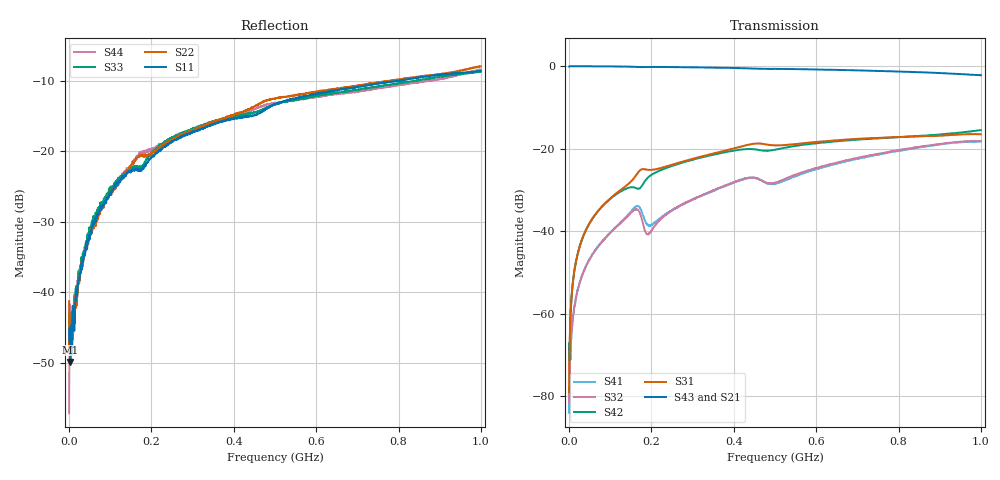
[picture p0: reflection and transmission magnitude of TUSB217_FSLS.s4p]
!Agilent Technologies,N5230A,US43500443,A.07.50.67
!Agilent N5230A: A.07.50.67
!Date: Wednesday, December 05, 2018 10:57:58
!Correction: S11(Full 4 Port(1,2,3,4))
!S12(Full 4 Port(1,2,3,4))
!S13(Full 4 Port(1,2,3,4))
!S14(Full 4 Port(1,2,3,4))
!S21(Full 4 Port(1,2,3,4))
!S22(Full 4 Port(1,2,3,4))
!S23(Full 4 Port(1,2,3,4))
!S24(Full 4 Port(1,2,3,4))
!S31(Full 4 Port(1,2,3,4))
!S32(Full 4 Port(1,2,3,4))
!S33(Full 4 Port(1,2,3,4))
!S34(Full 4 Port(1,2,3,4))
!S41(Full 4 Port(1,2,3,4))
!S42(Full 4 Port(1,2,3,4))
!S43(Full 4 Port(1,2,3,4))
!S44(Full 4 Port(1,2,3,4))
!S4P File: Measurements: <S11,S12,S13,S14>,
!<S21,S22,S23,S24>,
!<S31,S32,S33,S34>,
!<S41,S42,S43,S44>:
# Hz S  dB  R 50
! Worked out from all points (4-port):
!   1601 points, 300 kHz to 1 GHz, reference 50 ohm
!   strongest paths, dB at 300 kHz, 250.2 MHz, 500.1 MHz, 750.1 MHz, 1 GHz:
!     S43: -0.1, -0.2, -0.7, -1.2, -2.2
!     S21: -0.1, -0.2, -0.8, -1.2, -2.3
!     S31: -79.1, -23.9, -19.2, -17.4, -16.5
!     S42: -67.2, -24.2, -20.3, -17.5, -15.5
!     S32: -69.2, -35.0, -28.3, -21.3, -18.2
!     S41: -78.9, -34.9, -28.6, -21.5, -18.3
!   lowest |S11| = -49.9 dB at 3.424 MHz (marker M1), VSWR 1.01, Z = 50.3 - j0.118 ohm
!   |S11| at or under -10 dB: start of sweep to 798 MHz; 799.1297 MHz to 800.5317 MHz (1.402 MHz wide, 0.175 % of centre); 800.7341 MHz to 802.0164 MHz (1.282 MHz wide, 0.16 % of centre)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
300000  -46.87 -16.9  -0.09 0.9  -74.67 15.3  -73.35 -149.2
        -0.08 0.4  -41.25 -90.0  -82.33 -177.2  -80.37 70.3
        -79.12 -25.8  -69.18 -120.3  -47.18 -21.7  -0.12 1.4
        -78.88 136.5  -67.23 -114.8  -0.12 1.1  -57.15 40.3
3424062  -49.85 -21.4  -0.04 -0.1  -61.11 88.5  -69.45 -82.4
         -0.03 -0.2  -45.47 -17.6  -69.11 -87.3  -60.28 86.4
         -60.73 84.8  -71.22 -88.7  -48.24 -19.8  -0.03 -0.1
         -70.38 -91.1  -60.79 89.1  -0.04 -0.0  -45.54 -21.3
1.404588e7  -44.34 -65.5  -0.04 -0.9  -48.93 88.5  -57.65 -92.1
            -0.04 -1.0  -42.40 -48.8  -57.77 -91.7  -48.89 87.8
            -49.01 88.5  -57.96 -94.1  -42.76 -63.0  -0.04 -1.0
            -57.76 -92.1  -48.86 87.5  -0.04 -1.0  -41.97 -60.9
4.216244e7  -33.46 -80.3  -0.03 -2.8  -39.52 88.0  -48.32 -92.7
            -0.04 -2.9  -32.81 -78.7  -48.35 -92.3  -39.54 86.5
            -39.55 87.8  -48.34 -92.6  -32.71 -86.5  -0.05 -2.9
            -48.32 -92.5  -39.56 86.5  -0.06 -3.0  -33.21 -76.5
1.758723e8  -22.73 -105.4  -0.23 -11.6  -25.04 82.0  -35.29 -134.9
            -0.24 -11.7  -20.65 -97.1  -36.82 -139.7  -29.20 87.6
            -25.06 81.9  -36.82 -139.5  -22.18 -104.9  -0.23 -12.0
            -35.20 -133.3  -29.20 87.3  -0.26 -11.9  -20.15 -95.8
4.020544e8  -15.41 -122.7  -0.48 -26.6  -19.91 68.0  -28.21 -104.7
            -0.48 -26.6  -14.79 -108.5  -28.08 -102.7  -20.45 67.2
            -19.92 68.1  -28.09 -102.8  -15.09 -125.3  -0.45 -27.0
            -28.19 -105.2  -20.47 67.3  -0.48 -26.9  -14.99 -106.3
1e9  -8.59 -153.0  -2.35 -63.2  -16.52 55.3  -18.28 -150.2
     -2.31 -63.0  -7.95 -164.7  -18.12 -152.4  -15.51 64.6
     -16.53 55.0  -18.15 -152.3  -8.71 -160.2  -2.23 -65.6
     -18.29 -149.6  -15.54 64.4  -2.21 -65.3  -8.39 -167.5
